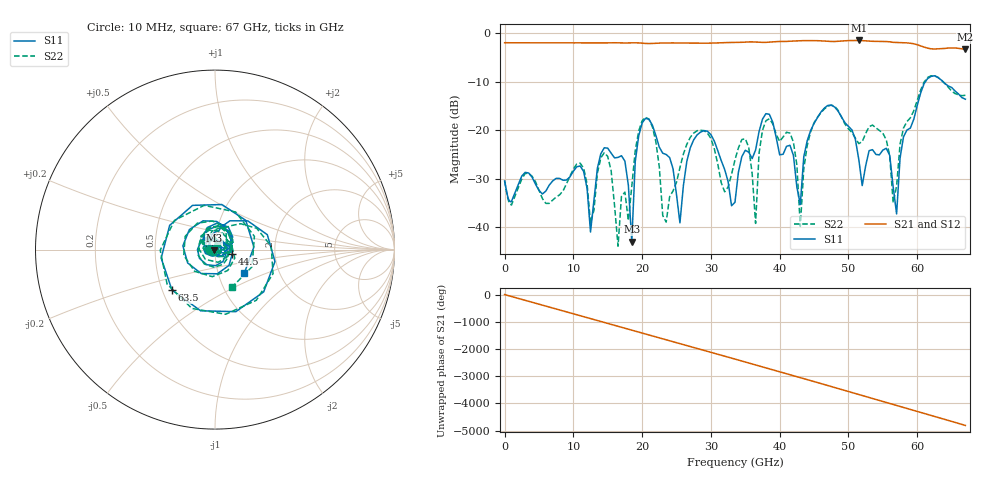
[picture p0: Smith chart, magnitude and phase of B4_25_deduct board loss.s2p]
!Keysight Technologies,N5247B,MY61255065,A.16.20.04
!Date: Monday, September 04, 2023 01:13:43
!Correction: S11(C  2-Port  )
!S21(C  2-Port  )
!S12(C  2-Port  )
!S22(C  2-Port  )
!S2P File: Measurements: S11, S21, S12, S22:
!Deduct Board Loss
# Hz S  dB  R 50
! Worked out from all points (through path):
!   142 points, 10 MHz to 67 GHz, reference 50 ohm
!   highest |S21| = -1.48 dB at 51.5 GHz (marker M1); lowest = -3.3 dB at 67 GHz (marker M2)
!   lowest |S11| = -43.0 dB at 18.5 GHz (marker M3), VSWR 1.01, Z = 49.5 - j0.445 ohm
!   |S11| at or under -10 dB: start of sweep to 61.18 GHz; 63.75 GHz to end of sweep
!   |S22| runs from -43.9 to -8.8 dB; largest |S21 - S12| = 0.0038
!   S11 on the Smith chart (normalised r, x): 10 MHz: 0.94, -0.00; 44.5 GHz: 1.21, -0.05; 63.5 GHz: 0.56, -0.28; 67 GHz: 1.33, -0.36
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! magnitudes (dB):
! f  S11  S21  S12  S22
! 10 MHz  -30.4  -2.0  -1.9  -30.4
! 11.5 GHz  -28.5  -2.0  -2.0  -27.8
! 12.5 GHz  -41.0  -2.0  -2.0  -39.2
! 14.5 GHz  -23.6  -2.0  -2.0  -24.6
! 17 GHz  -25.3  -2.0  -2.0  -33.6
! 18.5 GHz  -43.0  -2.0  -2.0  -31.6
! 20 GHz  -18.5  -2.0  -2.1  -18.0
! 22.5 GHz  -23.5  -2.0  -2.0  -27.6
! 25.5 GHz  -39.1  -2.0  -2.0  -27.7
! 28 GHz  -20.9  -2.0  -2.0  -20.1
! 34 GHz  -28.7  -1.9  -1.9  -23.6
! 36.5 GHz  -24.1  -1.8  -1.8  -39.2
! 38 GHz  -16.6  -1.9  -1.9  -18.0
! 41.5 GHz  -23.1  -1.6  -1.6  -20.6
! 43 GHz  -35.3  -1.5  -1.5  -39.8
! 44.5 GHz  -20.1  -1.5  -1.5  -20.3
! 45 GHz  -18.6  -1.5  -1.5  -18.4
! 51.5 GHz  -26.0  -1.5  -1.5  -22.7
! 56 GHz  -25.2  -1.8  -1.8  -25.3
! 57 GHz  -37.3  -1.9  -1.9  -31.5
! 63.5 GHz  -9.6  -3.2  -3.2  -9.7
! 67 GHz  -13.6  -3.3  -3.3  -12.8
